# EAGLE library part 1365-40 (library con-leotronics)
DUAL ROW STRAIGHT HEADER 1364 SERIES. 1.27mm x 1.27mm. Without Fixing Post. SMT Source: http://www.leotronics.co.uk/Conexcon/Data%20Sheets/sec.%20A/1364ing.pdf
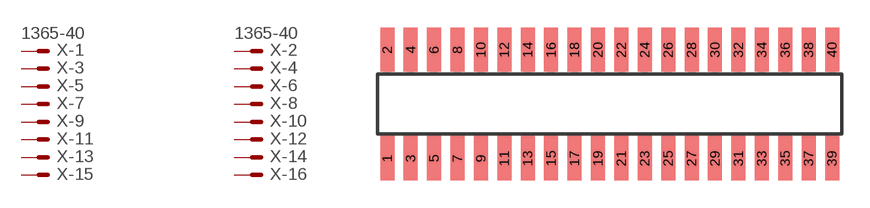
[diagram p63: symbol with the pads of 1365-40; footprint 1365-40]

Designator prefix X; gates -1=MVAL -2=MVAL -3=M -4=M -5=M -6=M -7=M -8=M -9=M -10=M -11=M -12=M -13=M -14=M -15=M -16=M -17=M -18=M -19=M -20=M -21=M -22=M -23=M -24=M -25=M -26=M -27=M -28=M -29=M -30=M -31=M -32=M -33=M -34=M -35=M -36=M -37=M -38=M -39=M -40=M

## 1365-40 (OC_FARNELL: unknown; OC_NEWARK: unknown)  [1365-40]
1  -1:S  pas
2  -2:S  pas
3  -3:S  pas
4  -4:S  pas
5  -5:S  pas
6  -6:S  pas
7  -7:S  pas
8  -8:S  pas
9  -9:S  pas
10  -10:S  pas
11  -11:S  pas
12  -12:S  pas
13  -13:S  pas
14  -14:S  pas
15  -15:S  pas
16  -16:S  pas
17  -17:S  pas
18  -18:S  pas
19  -19:S  pas
20  -20:S  pas
21  -21:S  pas
22  -22:S  pas
23  -23:S  pas
24  -24:S  pas
25  -25:S  pas
26  -26:S  pas
27  -27:S  pas
28  -28:S  pas
29  -29:S  pas
30  -30:S  pas
31  -31:S  pas
32  -32:S  pas
33  -33:S  pas
34  -34:S  pas
35  -35:S  pas
36  -36:S  pas
37  -37:S  pas
38  -38:S  pas
39  -39:S  pas
40  -40:S  pas

## Footprint 1365-40 (pad centres in mm)
DUAL ROW STRAIGHT HEADER 1364 SERIES. 1.27mm x 1.27mm. Without Fixing Post. SMT Source: http://www.leotronics.co.uk/Conexcon/Data%20Sheets/sec.%20A/1364ing.pdf
smd 0.76 x 2.4: 1 -12.065,-2.95; 2 -12.065,2.95; 3 -10.795,-2.95; 4 -10.795,2.95; 5 -9.525,-2.95; 6 -9.525,2.95; 7 -8.255,-2.95; 8 -8.255,2.95; 9 -6.985,-2.95; 10 -6.985,2.95; 11 -5.715,-2.95; 12 -5.715,2.95; 13 -4.445,-2.95; 14 -4.445,2.95; 15 -3.175,-2.95; 16 -3.175,2.95; 17 -1.905,-2.95; 18 -1.905,2.95; 19 -0.635,-2.95; 20 -0.635,2.95; 21 0.635,-2.95; 22 0.635,2.95; 23 1.905,-2.95; 24 1.905,2.95; 25 3.175,-2.95; 26 3.175,2.95; 27 4.445,-2.95; 28 4.445,2.95; 29 5.715,-2.95; 30 5.715,2.95; 31 6.985,-2.95; 32 6.985,2.95; 33 8.255,-2.95; 34 8.255,2.95; 35 9.525,-2.95; 36 9.525,2.95; 37 10.795,-2.95; 38 10.795,2.95; 39 12.065,-2.95; 40 12.065,2.95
